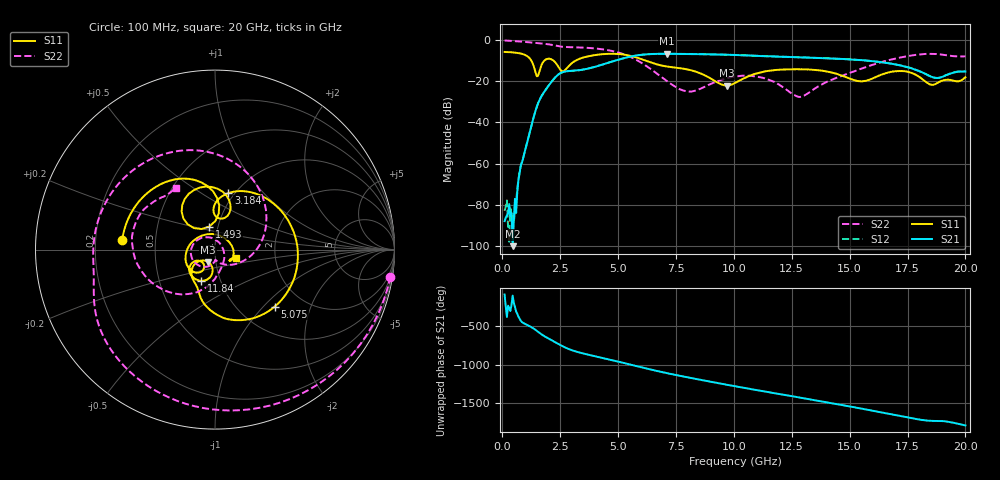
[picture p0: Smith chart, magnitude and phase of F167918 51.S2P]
!  2-Port S-parameters saved by WinCal
! VAR MeasName=S-Parameters (CALIBRATED_DATA) read from VNA (N5242A)
! VAR MeasDate=2016-11-22 10:27:17
! VAR NAME=F167918 51
! VAR FILENAME=F167918 51.S2P
! VAR DATE=2016-11-22 10:27:17
! VAR PHYS_PORTS=1,2
# Hz S DB R 50
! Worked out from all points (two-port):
!   401 points, 100 MHz to 20 GHz, reference 50 ohm
!   highest |S21| = -6.57 dB at 7.115 GHz (marker M1); lowest = -100.2 dB at 448.2 MHz (marker M2)
!   |S21| within 3 dB of the highest: 4.972 GHz to 15.39 GHz (10.42 GHz wide, 102 % of centre)
!   lowest |S11| = -22.1 dB at 9.702 GHz (marker M3), VSWR 1.17, Z = 45.8 - j6.33 ohm
!   |S11| at or under -10 dB: 1.258 GHz to 1.811 GHz (552.8 MHz wide, 36 % of centre); 2.216 GHz to 3.152 GHz (935.1 MHz wide, 34.8 % of centre); 6.218 GHz to end of sweep
!   |S22| runs from -27.6 to -0.1 dB; largest |S21 - S12| = 0.0038
!   S11 on the Smith chart (normalised r, x): 100 MHz: 0.32, +0.05; 1.493 GHz: 0.91, +0.24; 3.184 GHz: 0.94, +0.66; 5.075 GHz: 1.45, -1.16; 11.84 GHz: 0.81, -0.29; 20 GHz: 1.25, -0.12
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1e8  -5.68 174.1  -88.00 -100.9  -83.01 88.3  -0.10 -8.8
4.4825e8  -5.90 153.1  -100.20 -115.1  -84.57 -87.4  -0.33 -37.0
1.095e9  -7.88 106.1  -48.82 -135.2  -48.82 -134.9  -0.91 -84.5
1.493e9  -17.58 103.9  -32.28 152.3  -32.28 152.6  -1.33 -110.1
1.891e9  -9.28 115.1  -23.79 71.2  -23.79 71.3  -1.82 -133.3
2.33875e9  -11.51 71.2  -17.45 -1.9  -17.44 -1.8  -2.68 -156.5
3.1845e9  -9.79 76.6  -14.74 -112.9  -14.73 -113.0  -3.43 170.5
3.43325e9  -8.63 60.8  -14.39 -133.3  -14.38 -133.3  -3.53 159.7
5.075e9  -6.75 -43.6  -9.22 112.9  -9.23 112.9  -6.17 76.1
5.82125e9  -8.47 -84.5  -7.37 58.2  -7.35 58.2  -9.75 28.6
6.7665e9  -12.02 -111.5  -6.60 -8.2  -6.59 -8.2  -16.97 -34.4
7.11475e9  -12.78 -116.0  -6.57 -30.7  -6.57 -30.6  -19.94 -55.6
8.259e9  -14.92 -136.8  -6.72 -99.1  -6.71 -99.1  -24.80 -88.8
9.70175e9  -22.06 -119.5  -7.04 -179.7  -7.03 -179.7  -18.41 -128.5
1.005e10  -20.79 -102.6  -7.15 161.5  -7.16 161.5  -17.65 -142.9
1.1841e10  -14.46 -113.6  -7.96 67.7  -7.90 67.9  -20.78 131.3
1.278625e10  -14.13 -127.1  -8.30 19.2  -8.25 19.1  -27.53 39.4
1.338325e10  -14.37 -135.7  -8.52 -11.8  -8.47 -12.0  -24.42 -30.7
1.49255e10  -18.30 -149.0  -9.28 -93.5  -9.24 -93.8  -16.17 -88.5
1.67165e10  -15.60 -130.0  -11.22 165.9  -11.27 165.9  -9.58 -132.4
1.83085e10  -20.34 117.0  -16.61 81.4  -16.56 81.4  -6.64 173.1
2e10  -18.04 -22.9  -15.19 17.8  -15.11 18.0  -7.83 122.0
